(* Logix 5000 AddOnInstructionDefinition export ResetSign; software revision 17.00 *)

ADD_ON_INSTRUCTION ResetSign   (* revision 1.0, vendor Electronic Displays, Inc., ExecuteEnableInFalse *)
// Reset Sign
// Erases All
// Variable Memory
// Revision note:
// Original Release
// 11-01-2012
// c.elston
VAR_IN_OUT
   Address : STRING; {required}   // "00" = all signs "01" = address 01 "02" = address 02 etc...(see protocol)
END_VAR
VAR_OUTPUT
   EN : BOOL; {visible}   // Instruction Interface Enable Bit
   DN : BOOL; {visible}   // Instruction Interface Done Bit
   ER : BOOL; {visible}   // Instruction Interface Error Bit
   IP : BOOL; {visible}   // Instruction Interface InProcess Bit
END_VAR
VAR_IN_OUT
   map_SignInput : SINT[32]; {required}   // Ethernet/IP LEDSIGN.I Data I/O Mapping
   map_SignOutput : SINT[496]; {required}   // Ethernet/IP LEDSIGN.O Data I/O Mapping
   Packet1Sent : STRING; {required}   // The actual packet sent to the sign (Packet1)
   Packet2Sent : STRING; {required}   // The actual packet sent to the sign (Packet2)
   Packet3Sent : STRING; {required}   // The actual packet sent to the sign (Packet3)
END_VAR
VAR
   SEQ : DINT;   // Sequence Number
   OktoCycle : BOOL;   // Ok to Cycle
   InCycle : BOOL;   // Incycle
   Error : BOOL;   // Error
   Enabled : BOOL;   // Enable ON Bit
   Done : BOOL;   // Done
   Disabled : BOOL;   // Disabled OFF Bit
   SignETX : STRING := '^C';   // DO NOT EDIT = ^C
   SignFileLabel : STRING;
   SignSOH : STRING := '^A';   // DO NOT EDIT = ^A
   SignAddress : STRING;
   SignSTX : STRING := '^B';   // DO NOT EDIT = ^B
   SignNULL : STRING;
   SignResetMemoryCommand : STRING := 'CM';   // DO NOT EDIT = SM
   SignCommandCode : STRING := 'C';   // DO NOT EDIT = C
   TotalPacketCount : DINT[7];   // Total Character Count
   Select : DINT;   // Packet Array Select
   PacketMax : DINT := 82;   // Max Packet Count
   PacketCount : DINT[7];
   Packet6Offset : DINT;
   Packet5Offset : DINT;
   Packet4Offset : DINT;
   Packet3Offset : DINT;
   Packet2Offset : DINT;
   Packet1Offset : DINT;
   Packet : STRING[7];   // Packet Array to send to sign
END_VAR

ROUTINE EnableInFalse   (* ladder *)
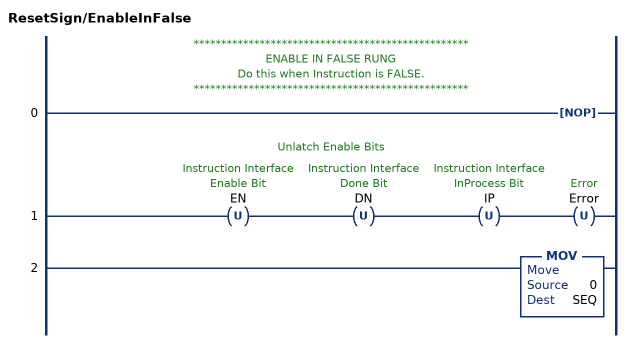
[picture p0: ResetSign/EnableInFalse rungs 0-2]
   // **************************************************
   // ENABLE IN FALSE RUNG
   // Do this when Instruction is FALSE.
   // **************************************************
   0: NOP();
   // Unlatch Enable Bits
   1: OTU(EN)OTU(DN)OTU(IP)OTU(Error);
   2: MOV(0,SEQ);
END_ROUTINE

ROUTINE Logic   (* ladder *)
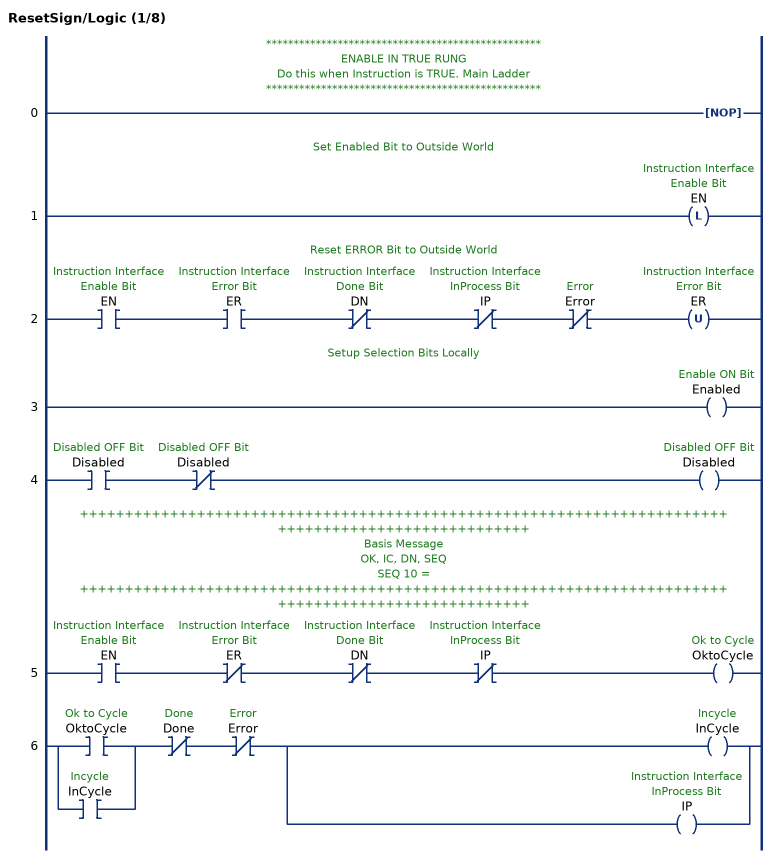
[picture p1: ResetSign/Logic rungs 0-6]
   // **************************************************
   // ENABLE IN TRUE RUNG
   // Do this when Instruction is TRUE. Main Ladder
   // **************************************************
   0: NOP();
   // Set Enabled Bit to Outside World
   1: OTL(EN);
   // Reset ERROR Bit to Outside World
   2: XIC(EN)XIC(ER)XIO(DN)XIO(IP)XIO(Error)OTU(ER);
   // Setup Selection Bits Locally
   3: OTE(Enabled);
   4: XIC(Disabled)XIO(Disabled)OTE(Disabled);
   // ++++++++++++++++++++++++++++++++++++++++++++++++++++++++++++++++++++++++++++++++++++++++++++++++++++
   // Basis Message
   // OK, IC, DN, SEQ
   // SEQ 10 =
   // ++++++++++++++++++++++++++++++++++++++++++++++++++++++++++++++++++++++++++++++++++++++++++++++++++++
   5: XIC(EN)XIO(ER)XIO(DN)XIO(IP)OTE(OktoCycle);
   6: [XIC(OktoCycle) ,XIC(InCycle) ]XIO(Done)XIO(Error)[OTE(InCycle) ,OTE(IP) ];
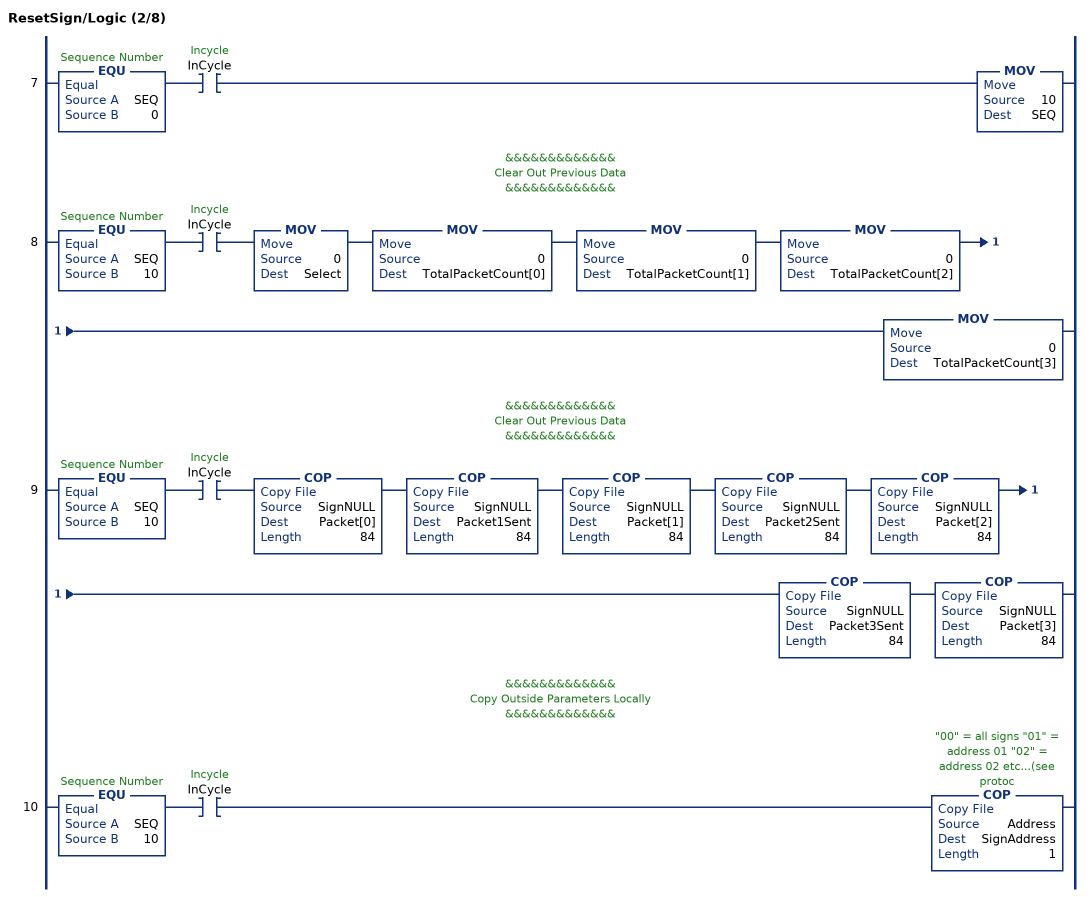
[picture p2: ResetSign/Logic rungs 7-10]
   7: EQU(SEQ,0)XIC(InCycle)MOV(10,SEQ);
   // &&&&&&&&&&&&&
   // Clear Out Previous Data
   // &&&&&&&&&&&&&
   8: EQU(SEQ,10)XIC(InCycle)MOV(0,Select)MOV(0,TotalPacketCount[0])MOV(0,TotalPacketCount[1])MOV(0,TotalPacketCount[2])MOV(0,TotalPacketCount[3]);
   // &&&&&&&&&&&&&
   // Clear Out Previous Data
   // &&&&&&&&&&&&&
   9: EQU(SEQ,10)XIC(InCycle)COP(SignNULL,Packet[0],84)COP(SignNULL,Packet1Sent,84)COP(SignNULL,Packet[1],84)COP(SignNULL,Packet2Sent,84)COP(SignNULL,Packet[2],84)COP(SignNULL,Packet3Sent,84)COP(SignNULL,Packet[3],84);
   // &&&&&&&&&&&&&
   // Copy Outside Parameters Locally
   // &&&&&&&&&&&&&
   10: EQU(SEQ,10)XIC(InCycle)COP(Address,SignAddress,1);
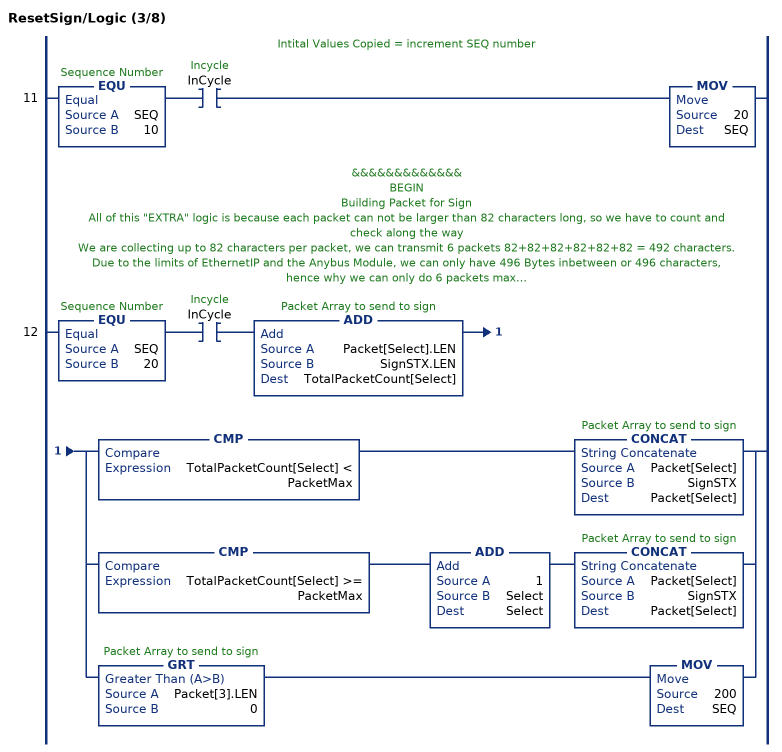
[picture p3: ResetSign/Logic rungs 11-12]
   // Intital Values Copied = increment SEQ number
   11: EQU(SEQ,10)XIC(InCycle)MOV(20,SEQ);
   // &&&&&&&&&&&&&
   // BEGIN
   // Building Packet for Sign
   // All of this "EXTRA" logic is because each packet can not be larger than 82 characters long, so we have to count and check along the way
   // We are collecting up to 82 characters per packet, we can transmit 6 packets 82+82+82+82+82+82 = 492 characters.
   // Due to the limits of EthernetIP and the Anybus Module, we can only have 496 Bytes inbetween or 496 characters, hence why we can only do 6 packets max.
   // Once we exceed this, we will fault and ERROR trap any windy typing people.
   // In this instruction below, it's so small, we are only using 3 packets max.
   // &&&&&&&&&&&&&
   12: EQU(SEQ,20)XIC(InCycle)ADD(Packet[Select].LEN,SignSTX.LEN,TotalPacketCount[Select])[CMP(TotalPacketCount[Select] < PacketMax) CONCAT(Packet[Select],SignSTX,Packet[Select]) ,CMP(TotalPacketCount[Select] >= PacketMax) ADD(1,Select,Select) CONCAT(Packet[Select],SignSTX,Packet[Select]) ,GRT(Packet[3].LEN,0) MOV(200,SEQ) ];
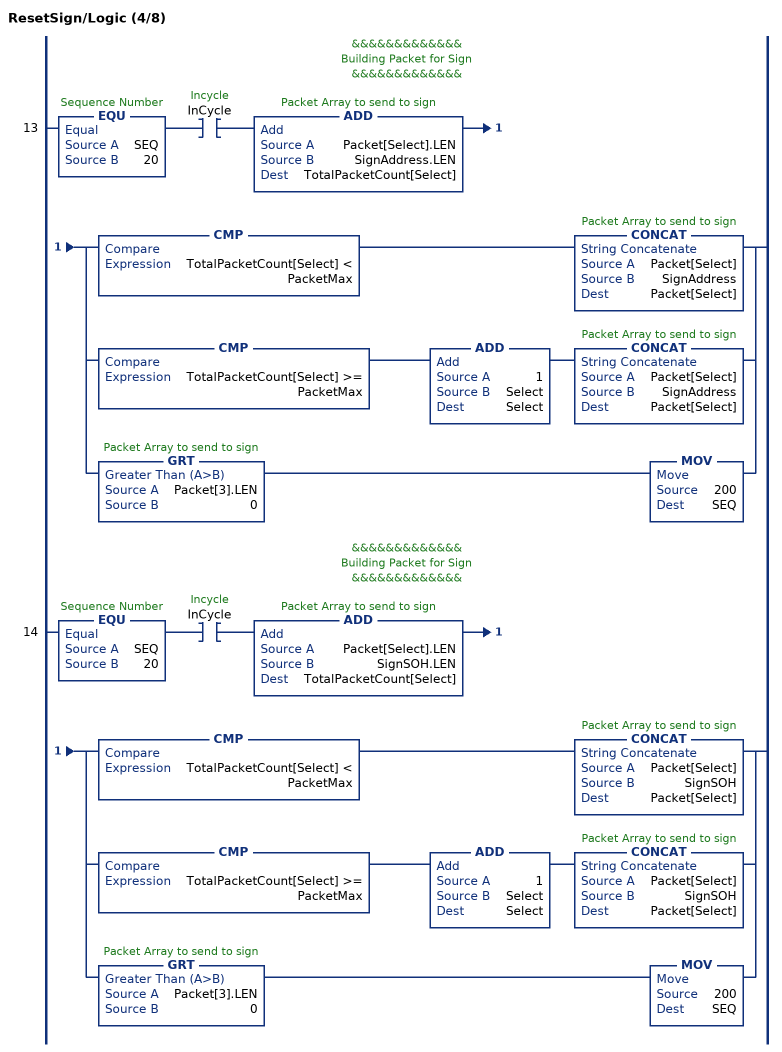
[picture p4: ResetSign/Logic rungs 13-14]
   // &&&&&&&&&&&&&
   // Building Packet for Sign
   // &&&&&&&&&&&&&
   13: EQU(SEQ,20)XIC(InCycle)ADD(Packet[Select].LEN,SignAddress.LEN,TotalPacketCount[Select])[CMP(TotalPacketCount[Select] < PacketMax) CONCAT(Packet[Select],SignAddress,Packet[Select]) ,CMP(TotalPacketCount[Select] >= PacketMax) ADD(1,Select,Select) CONCAT(Packet[Select],SignAddress,Packet[Select]) ,GRT(Packet[3].LEN,0) MOV(200,SEQ) ];
   // &&&&&&&&&&&&&
   // Building Packet for Sign
   // &&&&&&&&&&&&&
   14: EQU(SEQ,20)XIC(InCycle)ADD(Packet[Select].LEN,SignSOH.LEN,TotalPacketCount[Select])[CMP(TotalPacketCount[Select] < PacketMax) CONCAT(Packet[Select],SignSOH,Packet[Select]) ,CMP(TotalPacketCount[Select] >= PacketMax) ADD(1,Select,Select) CONCAT(Packet[Select],SignSOH,Packet[Select]) ,GRT(Packet[3].LEN,0) MOV(200,SEQ) ];
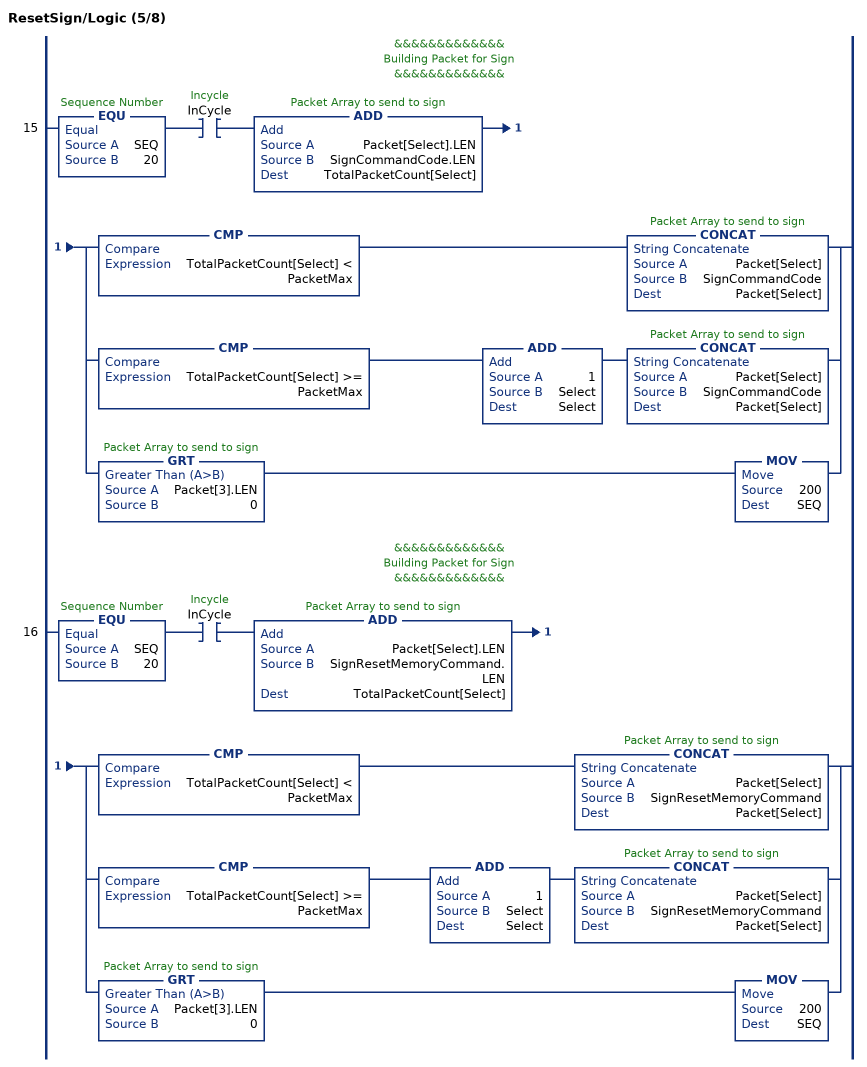
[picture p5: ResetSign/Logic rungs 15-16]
   // &&&&&&&&&&&&&
   // Building Packet for Sign
   // &&&&&&&&&&&&&
   15: EQU(SEQ,20)XIC(InCycle)ADD(Packet[Select].LEN,SignCommandCode.LEN,TotalPacketCount[Select])[CMP(TotalPacketCount[Select] < PacketMax) CONCAT(Packet[Select],SignCommandCode,Packet[Select]) ,CMP(TotalPacketCount[Select] >= PacketMax) ADD(1,Select,Select) CONCAT(Packet[Select],SignCommandCode,Packet[Select]) ,GRT(Packet[3].LEN,0) MOV(200,SEQ) ];
   // &&&&&&&&&&&&&
   // Building Packet for Sign
   // &&&&&&&&&&&&&
   16: EQU(SEQ,20)XIC(InCycle)ADD(Packet[Select].LEN,SignResetMemoryCommand.LEN,TotalPacketCount[Select])[CMP(TotalPacketCount[Select] < PacketMax) CONCAT(Packet[Select],SignResetMemoryCommand,Packet[Select]) ,CMP(TotalPacketCount[Select] >= PacketMax) ADD(1,Select,Select) CONCAT(Packet[Select],SignResetMemoryCommand,Packet[Select]) ,GRT(Packet[3].LEN,0) MOV(200,SEQ) ];
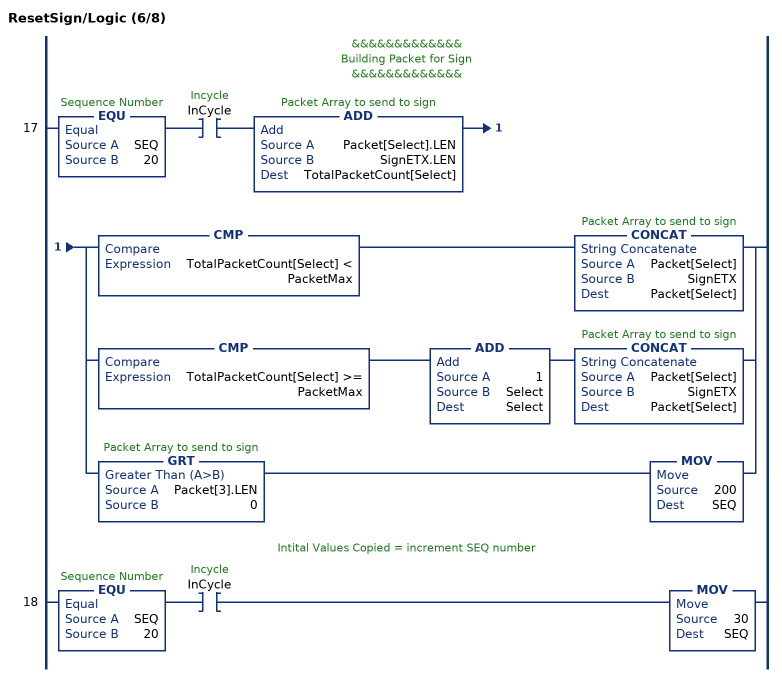
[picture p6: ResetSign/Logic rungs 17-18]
   // &&&&&&&&&&&&&
   // Building Packet for Sign
   // &&&&&&&&&&&&&
   17: EQU(SEQ,20)XIC(InCycle)ADD(Packet[Select].LEN,SignETX.LEN,TotalPacketCount[Select])[CMP(TotalPacketCount[Select] < PacketMax) CONCAT(Packet[Select],SignETX,Packet[Select]) ,CMP(TotalPacketCount[Select] >= PacketMax) ADD(1,Select,Select) CONCAT(Packet[Select],SignETX,Packet[Select]) ,GRT(Packet[3].LEN,0) MOV(200,SEQ) ];
   // Intital Values Copied = increment SEQ number
   18: EQU(SEQ,20)XIC(InCycle)MOV(30,SEQ);
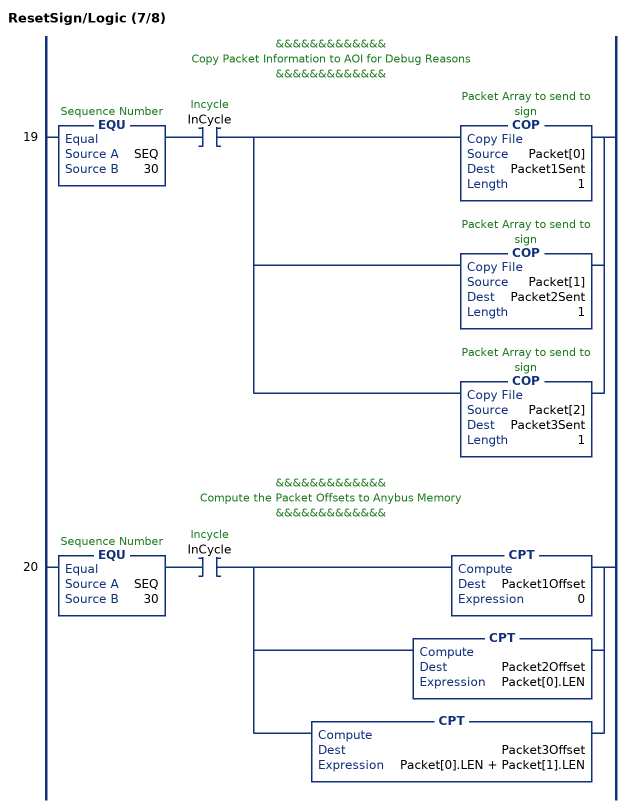
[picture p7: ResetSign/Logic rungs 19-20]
   // &&&&&&&&&&&&&
   // Copy Packet Information to AOI for Debug Reasons
   // &&&&&&&&&&&&&
   19: EQU(SEQ,30)XIC(InCycle)[COP(Packet[0],Packet1Sent,1) ,COP(Packet[1],Packet2Sent,1) ,COP(Packet[2],Packet3Sent,1) ];
   // &&&&&&&&&&&&&
   // Compute the Packet Offsets to Anybus Memory
   // &&&&&&&&&&&&&
   20: EQU(SEQ,30)XIC(InCycle)[CPT(Packet1Offset,0) ,CPT(Packet2Offset,Packet[0].LEN) ,CPT(Packet3Offset,Packet[0].LEN + Packet[1].LEN) ];
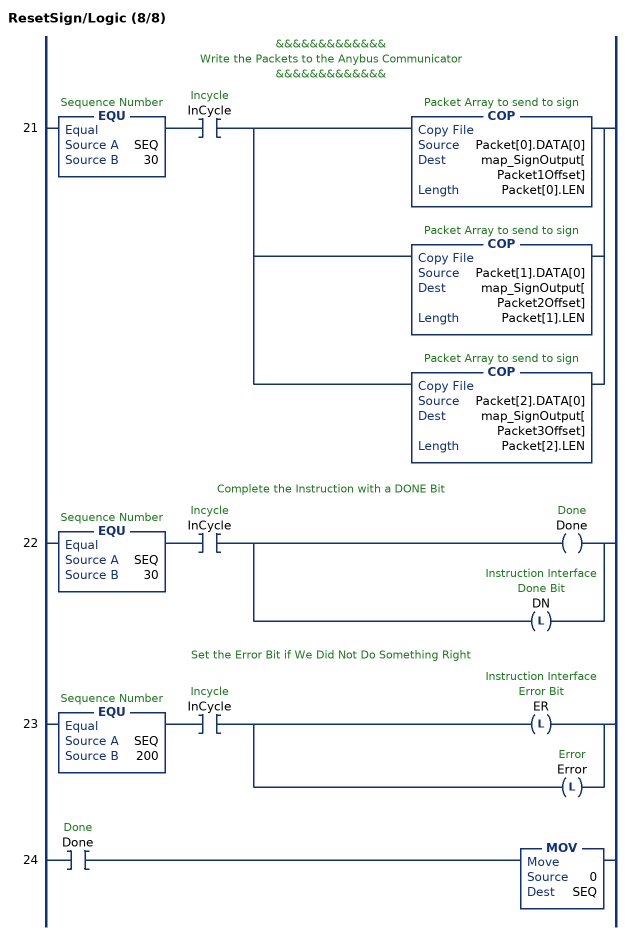
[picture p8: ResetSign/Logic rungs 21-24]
   // &&&&&&&&&&&&&
   // Write the Packets to the Anybus Communicator
   // &&&&&&&&&&&&&
   21: EQU(SEQ,30)XIC(InCycle)[COP(Packet[0].DATA[0],map_SignOutput[Packet1Offset],Packet[0].LEN) ,COP(Packet[1].DATA[0],map_SignOutput[Packet2Offset],Packet[1].LEN) ,COP(Packet[2].DATA[0],map_SignOutput[Packet3Offset],Packet[2].LEN) ];
   // Complete the Instruction with a DONE Bit
   22: EQU(SEQ,30)XIC(InCycle)[OTE(Done) ,OTL(DN) ];
   // Set the Error Bit if We Did Not Do Something Right
   23: EQU(SEQ,200)XIC(InCycle)[OTL(ER) ,OTL(Error) ];
   24: XIC(Done)MOV(0,SEQ);
END_ROUTINE
END_ADD_ON_INSTRUCTION
